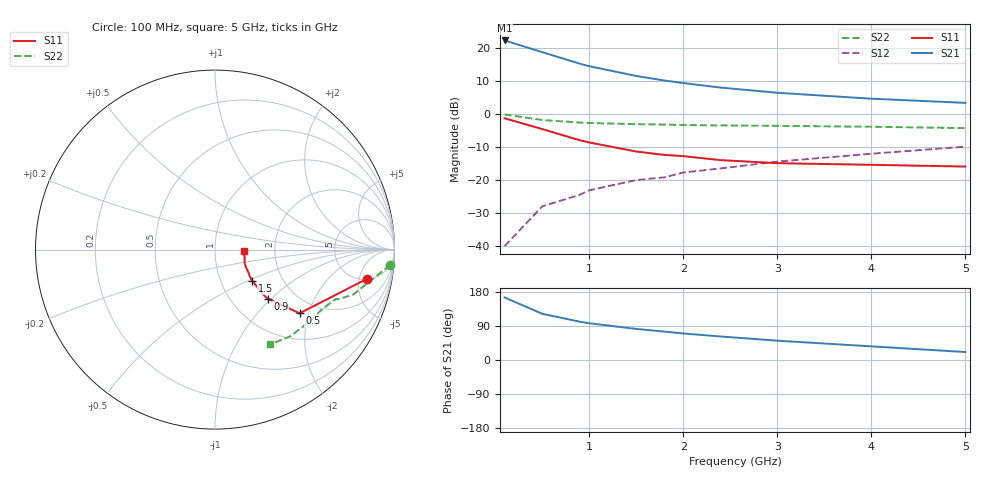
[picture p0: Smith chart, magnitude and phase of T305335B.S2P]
!AT-30533
!S and NOISE PARAMETERS at Vce=5V  Ic=5mA.  LAST UPDATED 04-10-94
# ghz s ma r 50!
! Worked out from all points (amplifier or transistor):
!   11 points, 100 MHz to 5 GHz, reference 50 ohm
!   highest |S21| = 22.2 dB at 100 MHz (marker M1)
!   |S21| within 3 dB of that: start of sweep to 439.4 MHz
!   unconditionally stable (mu >= 1): 1.667 GHz to 3.199 GHz
!   at 500 MHz: K = 0.67, MSG = 23.3 dB, |S12| = -28.0 dB
!   at 1.8 GHz: K = 1.02, MAG = 13.7 dB, |S12| = -19.2 dB
!   at 5 GHz: K = 0.95, MSG = 6.6 dB, |S12| = -9.9 dB
!   lowest NFmin = 1.10 dB at 500 MHz
!   S11 on the Smith chart (normalised r, x): 100 MHz: 5.09, -6.41; 500 MHz: 1.61, -1.75; 900 MHz: 1.46, -0.95; 1.5 GHz: 1.41, -0.53; 5 GHz: 1.38, -0.02
0.1  0.86 -11.0  12.92 165.0  0.01 83.0  0.98 -5.0
0.5  0.59 -37.0  8.6 122.0  0.04 72.0  0.81 -18.0
0.9  0.4 -43.0  5.75 101.0  0.06 70.0  0.74 -22.0
1  0.37 -43.0  5.27 97.0  0.07 70.0  0.73 -22.0
1.5  0.27 -40.0  3.75 82.0  0.1 68.0  0.7 -26.0
1.8  0.24 -37.0  3.2 75.0  0.11 67.0  0.69 -28.0
2  0.23 -35.0  2.93 70.0  0.13 66.0  0.68 -30.0
2.4  0.2 -30.0  2.5 62.0  0.15 64.0  0.67 -33.0
3  0.18 -24.0  2.09 51.0  0.19 61.0  0.66 -38.0
4  0.17 -14.0  1.7 36.0  0.25 54.0  0.64 -49.0
5  0.16 -2.0  1.47 21.0  0.32 46.0  0.61 -60.0
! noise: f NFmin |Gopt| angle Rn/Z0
0.5  1.1  0.71  8  0.78
0.9  1.2  0.61  16  0.66
1.8  1.5  0.42  39  0.41
2.4  1.8  0.28  57  0.25
